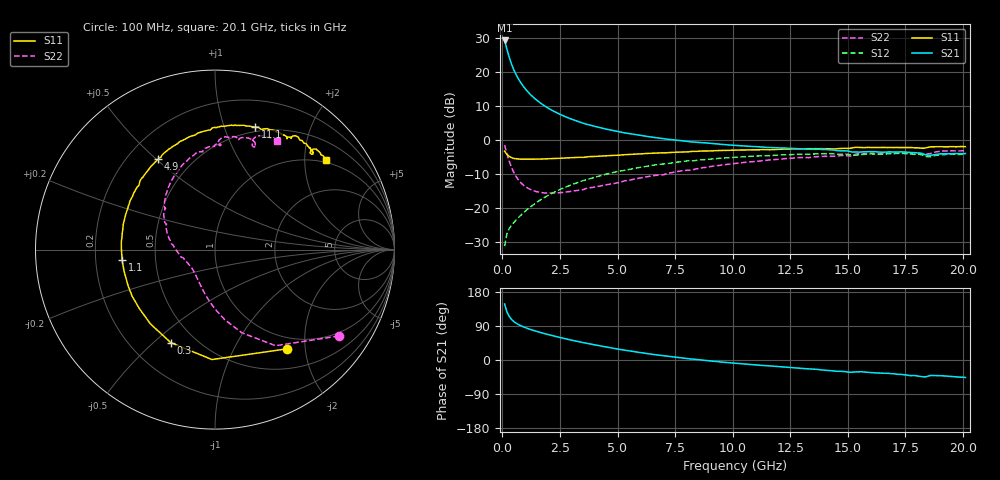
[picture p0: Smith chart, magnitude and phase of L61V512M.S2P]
!  Infineon Technologies AG
! BFR380L3 , PF131585-7, No.6, Th 09.10.01, soldered on pcb-board, measured with PP GSG850
!  Vce=1.5 V,  Ic=12.5 mA
! Common Emitter S-Parameters:  15. November 2001
#  GHz  S  MA  R  50
! f  S11  S21  S12  S22
! GHz  Mag  Ang  Mag  Ang  Mag  Ang  Mag  Ang
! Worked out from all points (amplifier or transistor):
!   201 points, 100 MHz to 20.1 GHz, reference 50 ohm
!   highest |S21| = 29.3 dB at 100 MHz (marker M1)
!   |S21| within 3 dB of that: start of sweep to 218.2 MHz
!   unconditionally stable (mu >= 1): 1.602 GHz to 4.818 GHz
!   at 3.4 GHz: K = 1.03, MAG = 7.7 dB, |S12| = -12.2 dB
!   at 10.1 GHz: K = 0.96, MSG = 1.7 dB, |S12| = -5.1 dB
!   at 20.1 GHz: K = 0.99, MSG = 0.1 dB, |S12| = -4.2 dB
!   S11 on the Smith chart (normalised r, x): 100 MHz: 0.80, -1.66; 300 MHz: 0.37, -0.57; 1.1 GHz: 0.32, -0.05; 4.9 GHz: 0.32, +0.51; 11.1 GHz: 0.45, +1.28; 20.1 GHz: 0.94, +2.54
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0.1  0.6831 -54.1  29.18 147.6  0.02734 65.4  0.8412 -34.9
0.2  0.6127 -91.6  21.71 127.0  0.04154 54.6  0.633 -57.8
0.3  0.5738 -115.4  16.5 114.9  0.04946 50.1  0.4869 -72.1
0.4  0.5484 -131.0  13.1 107.1  0.05545 49.2  0.3936 -82.1
0.5  0.5344 -142.0  10.78 101.4  0.06095 50.1  0.3317 -89.9
0.6  0.5298 -150.4  9.129 97.2  0.06645 51.2  0.2893 -96.2
0.7  0.5249 -157.0  7.92 93.5  0.07193 52.3  0.2584 -101.7
0.8  0.5211 -162.0  6.982 90.5  0.07765 53.8  0.2359 -106.5
0.9  0.5208 -166.6  6.242 87.9  0.08354 54.8  0.2185 -110.8
1.1  0.5207 -173.8  5.163 83.2  0.09587 56.5  0.1962 -118.5
1.3  0.5211 -179.9  4.399 79.0  0.1084 57.7  0.1817 -124.9
1.5  0.5236 174.9  3.841 75.3  0.121 58.3  0.173 -130.5
2  0.5307 164.3  2.928 67.0  0.1537 58.4  0.1655 -142.2
2.7  0.5416 151.9  2.228 56.6  0.1997 56.4  0.1709 -155.3
3.5  0.5549 139.9  1.772 46.0  0.2519 52.6  0.1848 -166.0
4.9  0.5947 122.3  1.355 30.1  0.3371 44.3  0.2306 175.1
6.8  0.6455 102.5  1.064 12.5  0.4372 31.5  0.3049 153.1
10.1  0.7091 77.7  0.8326 -8.5  0.557 10.2  0.4511 122.9
11.1  0.7182 71.7  0.7933 -13.5  0.582 3.9  0.4876 114.5
13.5  0.7426 60.2  0.7325 -24.1  0.6201 -10.2  0.5603 96.4
16.8  0.7757 48.0  0.6704 -35.3  0.6247 -25.9  0.6429 76.0
20.1  0.7961 38.7  0.6321 -46.3  0.6178 -39.3  0.695 60.3
